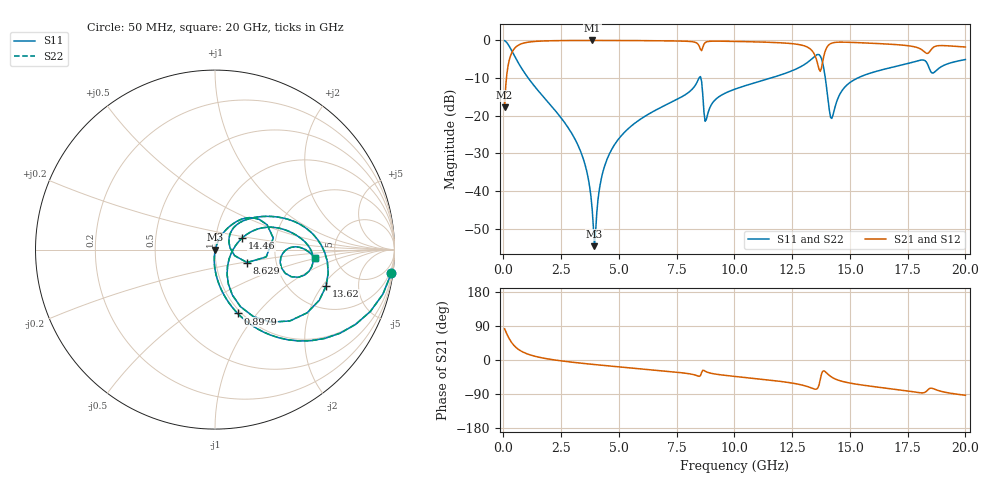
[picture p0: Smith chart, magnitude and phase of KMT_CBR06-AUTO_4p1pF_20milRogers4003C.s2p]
! Data measured by Modelithics Inc. support@modelithics.com 813-866-6335
! KEMET CBR06-AUTO 4.1pF, Pad Width= 0.851mm, Pad Length= 0.64mm, Pad Gap= 0.62mm, 20mil Rogers 4003C substrate Data, January 2022
# hz S ma R 50
! 2 Port Network Data from SP1.SP block
! freq  magS11  angS11  magS21  angS21  magS12  angS12  magS22  angS22
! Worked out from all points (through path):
!   401 points, 50 MHz to 20 GHz, reference 50 ohm
!   highest |S21| = -0.02 dB at 3.841 GHz (marker M1); lowest = -17.8 dB at 50 MHz (marker M2)
!   group delay of S21, straight-line fit = 15.2 ps
!   lowest |S11| = -54.6 dB at 3.94 GHz (marker M3), VSWR 1.00, Z = 50.2 - j0.0703 ohm
!   |S11| at or under -10 dB: 1.073 GHz to 8.468 GHz (7.395 GHz wide, 155 % of centre); 8.545 GHz to 11.57 GHz (3.023 GHz wide, 30.1 % of centre); 13.93 GHz to 15.33 GHz (1.396 GHz wide, 9.54 % of centre)
!   |S22| runs from -54.6 to -0.1 dB; largest |S21 - S12| = 0
!   S11 on the Smith chart (normalised r, x): 50 MHz: 1, -15; 897.9 MHz: 0.96, -0.80; 8.629 GHz: 1.42, -0.21; 13.62 GHz: 3.09, -2.18; 14.46 GHz: 1.34, +0.18; 20 GHz: 3.45, -0.44
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5e7  0.9916 -7.5  0.1287 82.4  0.1287 82.4  0.9916 -7.5
3.4925e8  0.7379 -43.4  0.674 46.5  0.674 46.5  0.7379 -43.4
8.97875e8  0.3772 -70.4  0.9251 19.4  0.9251 19.4  0.3772 -70.4
3.391625e9  0.03058 -95.4  0.9977 -8.6  0.9977 -8.6  0.03058 -95.4
3.690875e9  0.01365 -93.0  0.998 -10.5  0.998 -10.5  0.01365 -93.0
3.8405e9  0.005809 -83.3  0.998 -11.4  0.998 -11.4  0.005809 -83.3
3.94025e9  0.001857 -22.2  0.998 -12.0  0.998 -12.0  0.001857 -22.2
4.289375e9  0.01716 69.6  0.9978 -14.1  0.9978 -14.1  0.01716 69.6
4.688375e9  0.03581 70.5  0.9972 -16.3  0.9972 -16.3  0.03581 70.5
6.73325e9  0.1251 61.1  0.9892 -27.7  0.9892 -27.7  0.1251 61.1
8.478875e9  0.3215 25.6  0.8369 -43.1  0.8369 -43.1  0.3215 25.6
8.6285e9  0.1928 -21.9  0.8076 -27.2  0.8076 -27.2  0.1928 -21.9
8.778125e9  0.08787 28.0  0.9514 -30.9  0.9514 -30.9  0.08787 28.0
1.0025e10  0.2255 45.4  0.969 -43.3  0.969 -43.3  0.2255 45.4
1.336662e10  0.5744 5.6  0.7263 -74.6  0.7263 -74.6  0.5744 5.6
1.3616e10  0.6513 -18.2  0.4715 -73.1  0.4715 -73.1  0.6513 -18.2
1.38155e10  0.5094 -52.5  0.509 -30.4  0.509 -30.4  0.5094 -52.5
1.416462e10  0.09492 -34.8  0.9055 -43.3  0.9055 -43.3  0.09492 -34.8
1.446388e10  0.165 23.1  0.9458 -52.6  0.9458 -52.6  0.165 23.1
1.670825e10  0.4308 13.2  0.8911 -75.4  0.8911 -75.4  0.4308 13.2
1.835412e10  0.4898 -18.3  0.6703 -80.2  0.6703 -80.2  0.4898 -18.3
2e10  0.5571 -4.6  0.8163 -93.2  0.8163 -93.2  0.5571 -4.6
